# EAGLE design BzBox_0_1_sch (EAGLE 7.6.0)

## Sheet 1 of 6: BME280 EnvSense
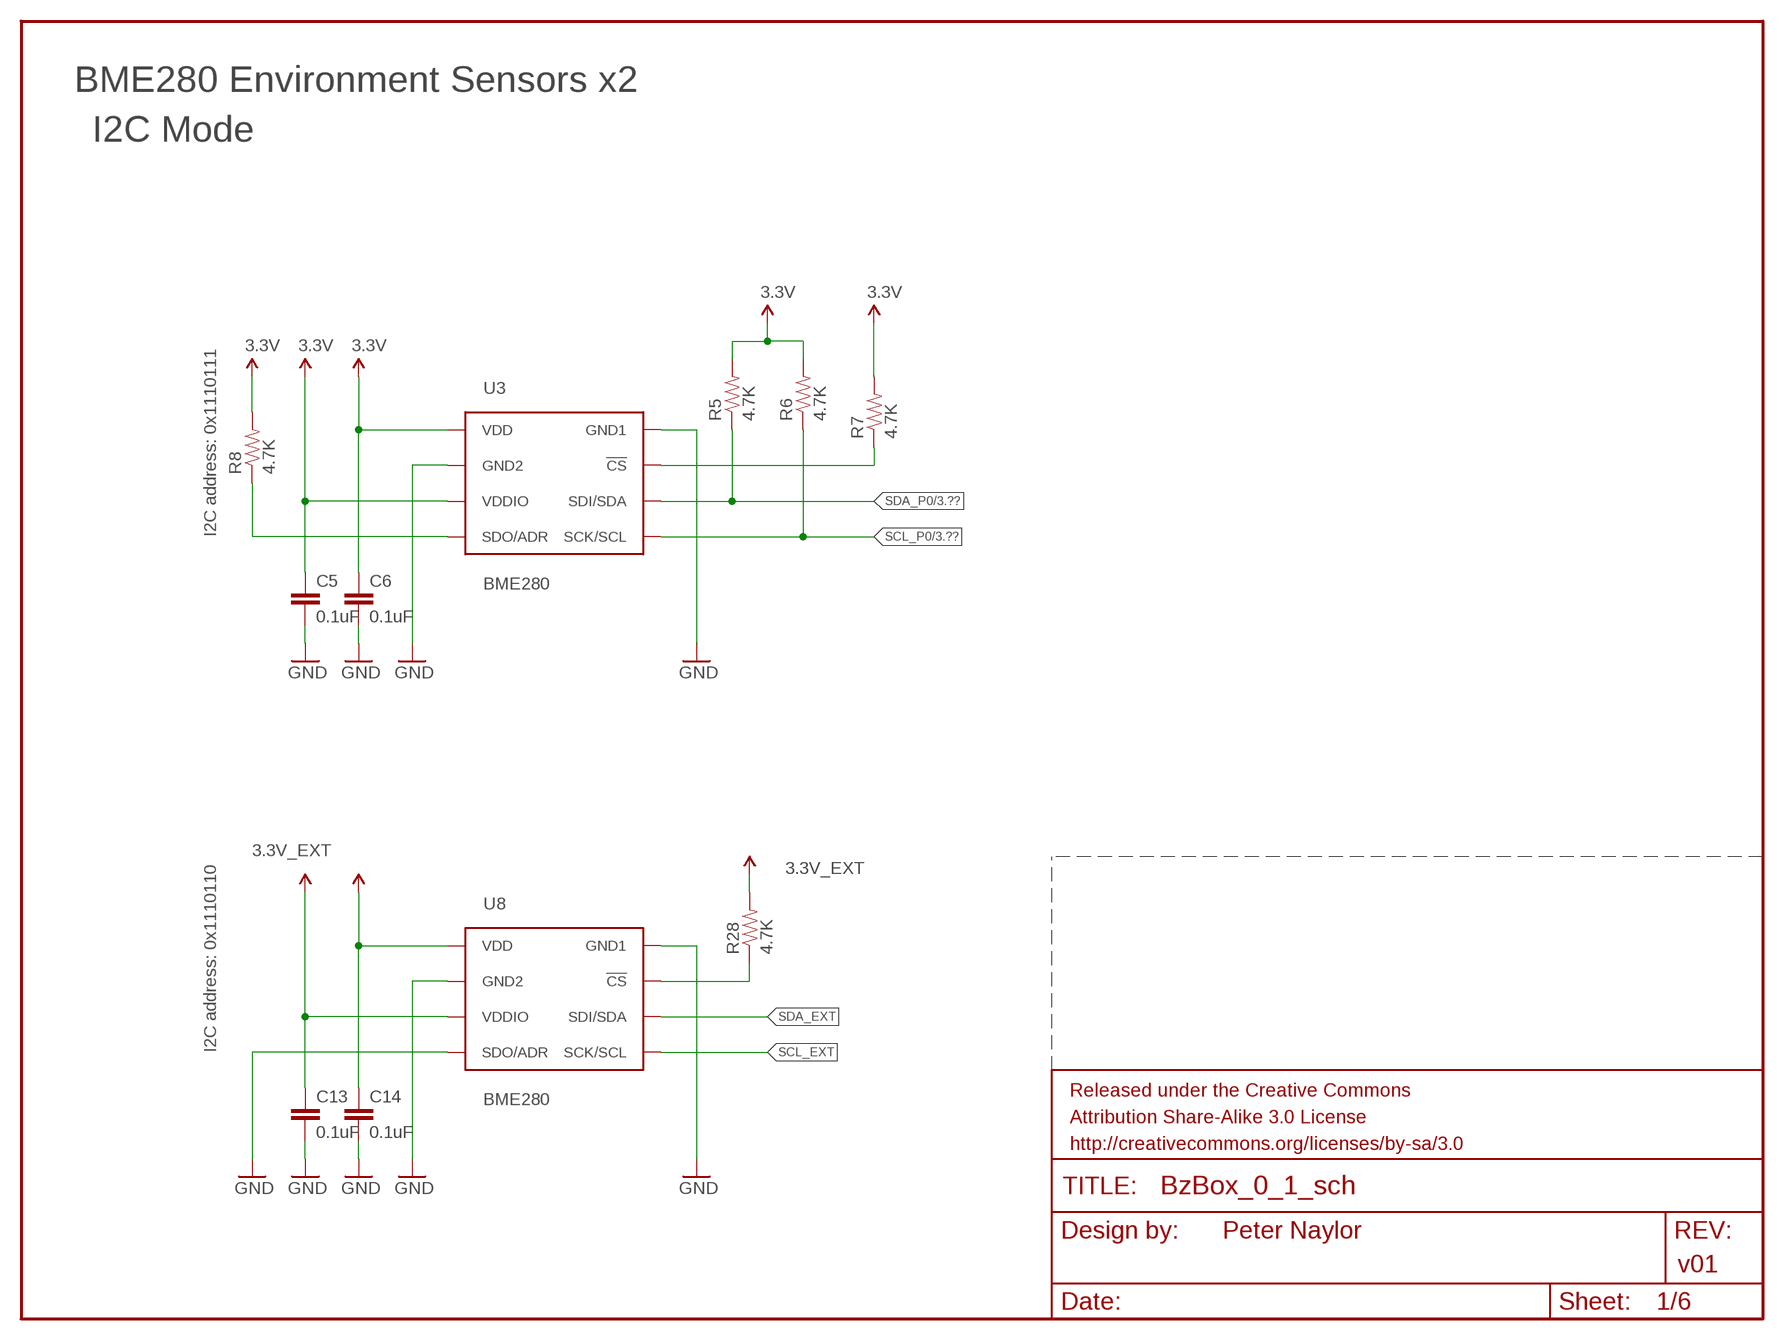
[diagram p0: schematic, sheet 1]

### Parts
C5  0.1uF  0.1UF-25V-5%(0603)  [0603-CAP@1]
C6  0.1uF  0.1UF-25V-5%(0603)  [0603-CAP@1]
C13  0.1uF  0.1UF-25V-5%(0603)  [0603-CAP@1]
C14  0.1uF  0.1UF-25V-5%(0603)  [0603-CAP@1]
R5  4.7K  4.7KOHM-1/10W-1%(0603)  [0603-RES]
R6  4.7K  4.7KOHM-1/10W-1%(0603)  [0603-RES]
R7  4.7K  4.7KOHM-1/10W-1%(0603)  [0603-RES]
R8  4.7K  4.7KOHM-1/10W-1%(0603)  [0603-RES]
R28  4.7K  4.7KOHM-1/10W-1%(0603)  [0603-RES]
U3  BME280  [BME280_LGA]
U8  BME280  [BME280_LGA]

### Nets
3.3V: C5.1 C6.1 R5.2 R6.2 R7.2 R8.2 U3.P$6(VDDIO) U3.P$8(VDD) ; also sheet 4,5,6
3.3V_EXT: C13.1 C14.1 R28.2 U8.P$6(VDDIO) U8.P$8(VDD) ; supply symbol labelled 3.3V ; also sheet 2
!CS: R7.1 U3.P$2(!CS)
GND: C5.2 C6.2 U3.P$1(GND1) U3.P$7(GND2) ; also sheet 3,4,5,6
GND_EXT: C13.2 C14.2 U8.P$1(GND1) U8.P$5(SDO/ADR) U8.P$7(GND2) ; supply symbol labelled GND ; also sheet 2
N$3: R28.1 U8.P$2(!CS)
SCL_EXT: U8.P$4(SCK/SCL) ; also sheet 2
SCL_P0: R6.1 U3.P$4(SCK/SCL) ; also sheet 3,5,6
SDA_EXT: U8.P$3(SDI/SDA) ; also sheet 2
SDA_P0: R5.1 U3.P$3(SDI/SDA) ; also sheet 3,5,6
SDO/ADR: R8.1 U3.P$5(SDO/ADR)

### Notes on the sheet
- BME280 Environment Sensors x2
- I2C Mode
- I2C address: 0x1110111
- I2C address: 0x1110110
- Peter Naylor
- v01

## Sheet 2 of 6: ADMP401 uPhone
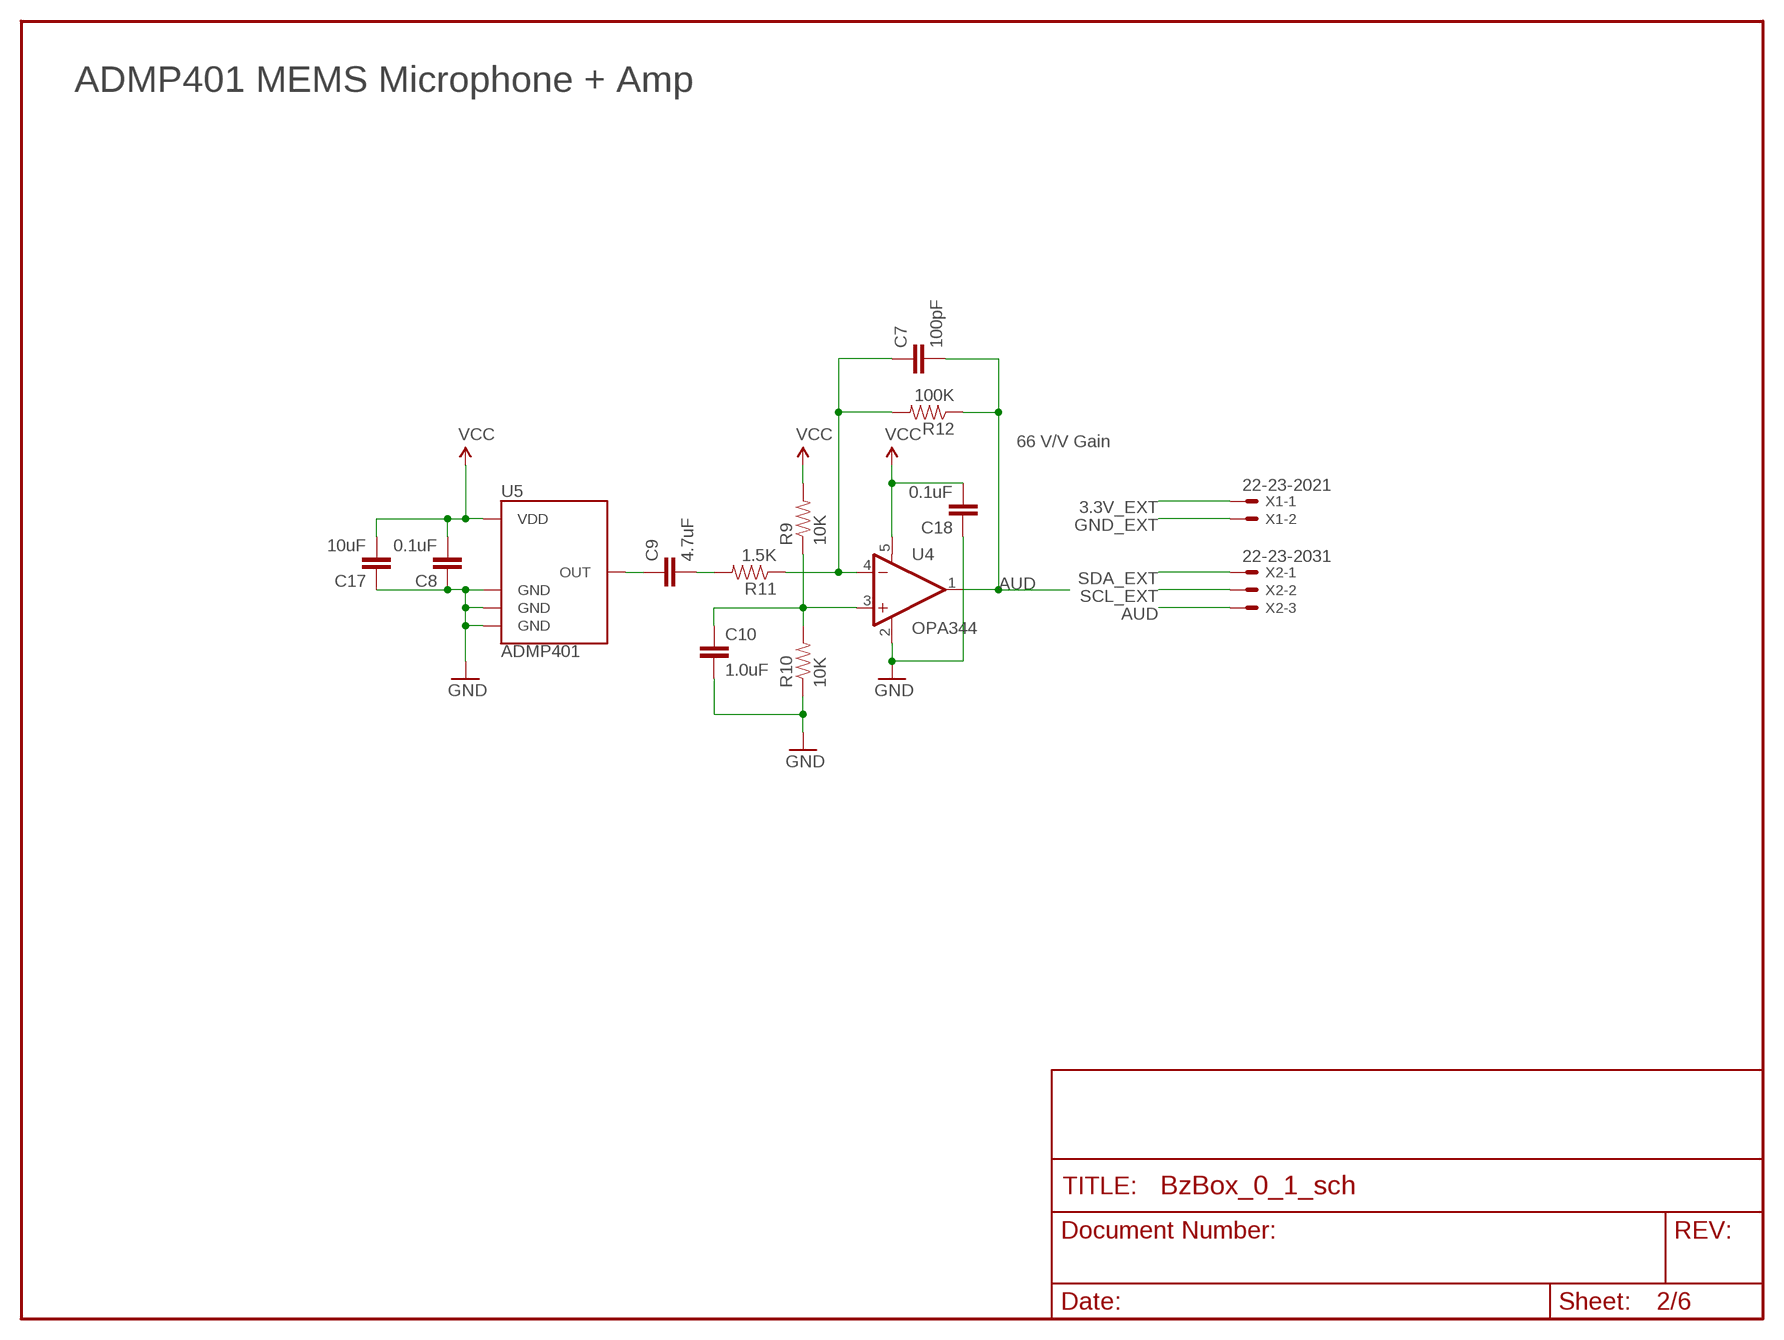
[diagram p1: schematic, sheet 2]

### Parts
C7  100pF  CAP0402-CAP  [0402-CAP]
C8  0.1uF  CAP0402-CAP  [0402-CAP]
C9  4.7uF  CAP0402-CAP  [0402-CAP]
C10  1.0uF  CAP0402-CAP  [0402-CAP]
C17  10uF  CAP0402-CAP  [0402-CAP]
C18  0.1uF  CAP0402-CAP  [0402-CAP]
R9  10K  RESISTOR0402-RES  [0402-RES]
R10  10K  RESISTOR0402-RES  [0402-RES]
R11  1.5K  RESISTOR0402-RES  [0402-RES]
R12  100K  RESISTOR0402-RES  [0402-RES]
U4  OPA344  [SOT23-5]
U5  ADMP401  [ADMP401]
X1  22-23-2021  [22-23-2021]
X2  22-23-2031  [22-23-2031]

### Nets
3.3V_EXT: C8.2 C17.2 C18.2 R9.2 U4.5(V+) U5.5(VDD) X1.1 ; supply symbol labelled VCC ; also sheet 1
AUD: C7.2 R12.1 U4.1(OUT) X2.3
GND_EXT: C8.1 C10.2 C17.1 C18.1 R10.1 U4.2(V-) U5.2(GND) U5.4(GND) U5.6(GND) X1.2 ; supply symbol labelled GND ; also sheet 1
N$9: C9.1 U5.1(OUT)
N$10: C7.1 R11.1 R12.2 U4.4(-IN)
N$11: C9.2 R11.2
N$12: C10.1 R9.1 R10.2 U4.3(+IN)
SCL_EXT: X2.2 ; also sheet 1
SDA_EXT: X2.1 ; also sheet 1

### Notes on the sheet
- ADMP401 MEMS Microphone + Amp
- 66 V/V Gain

## Sheet 3 of 6: Solar-Battery Charger
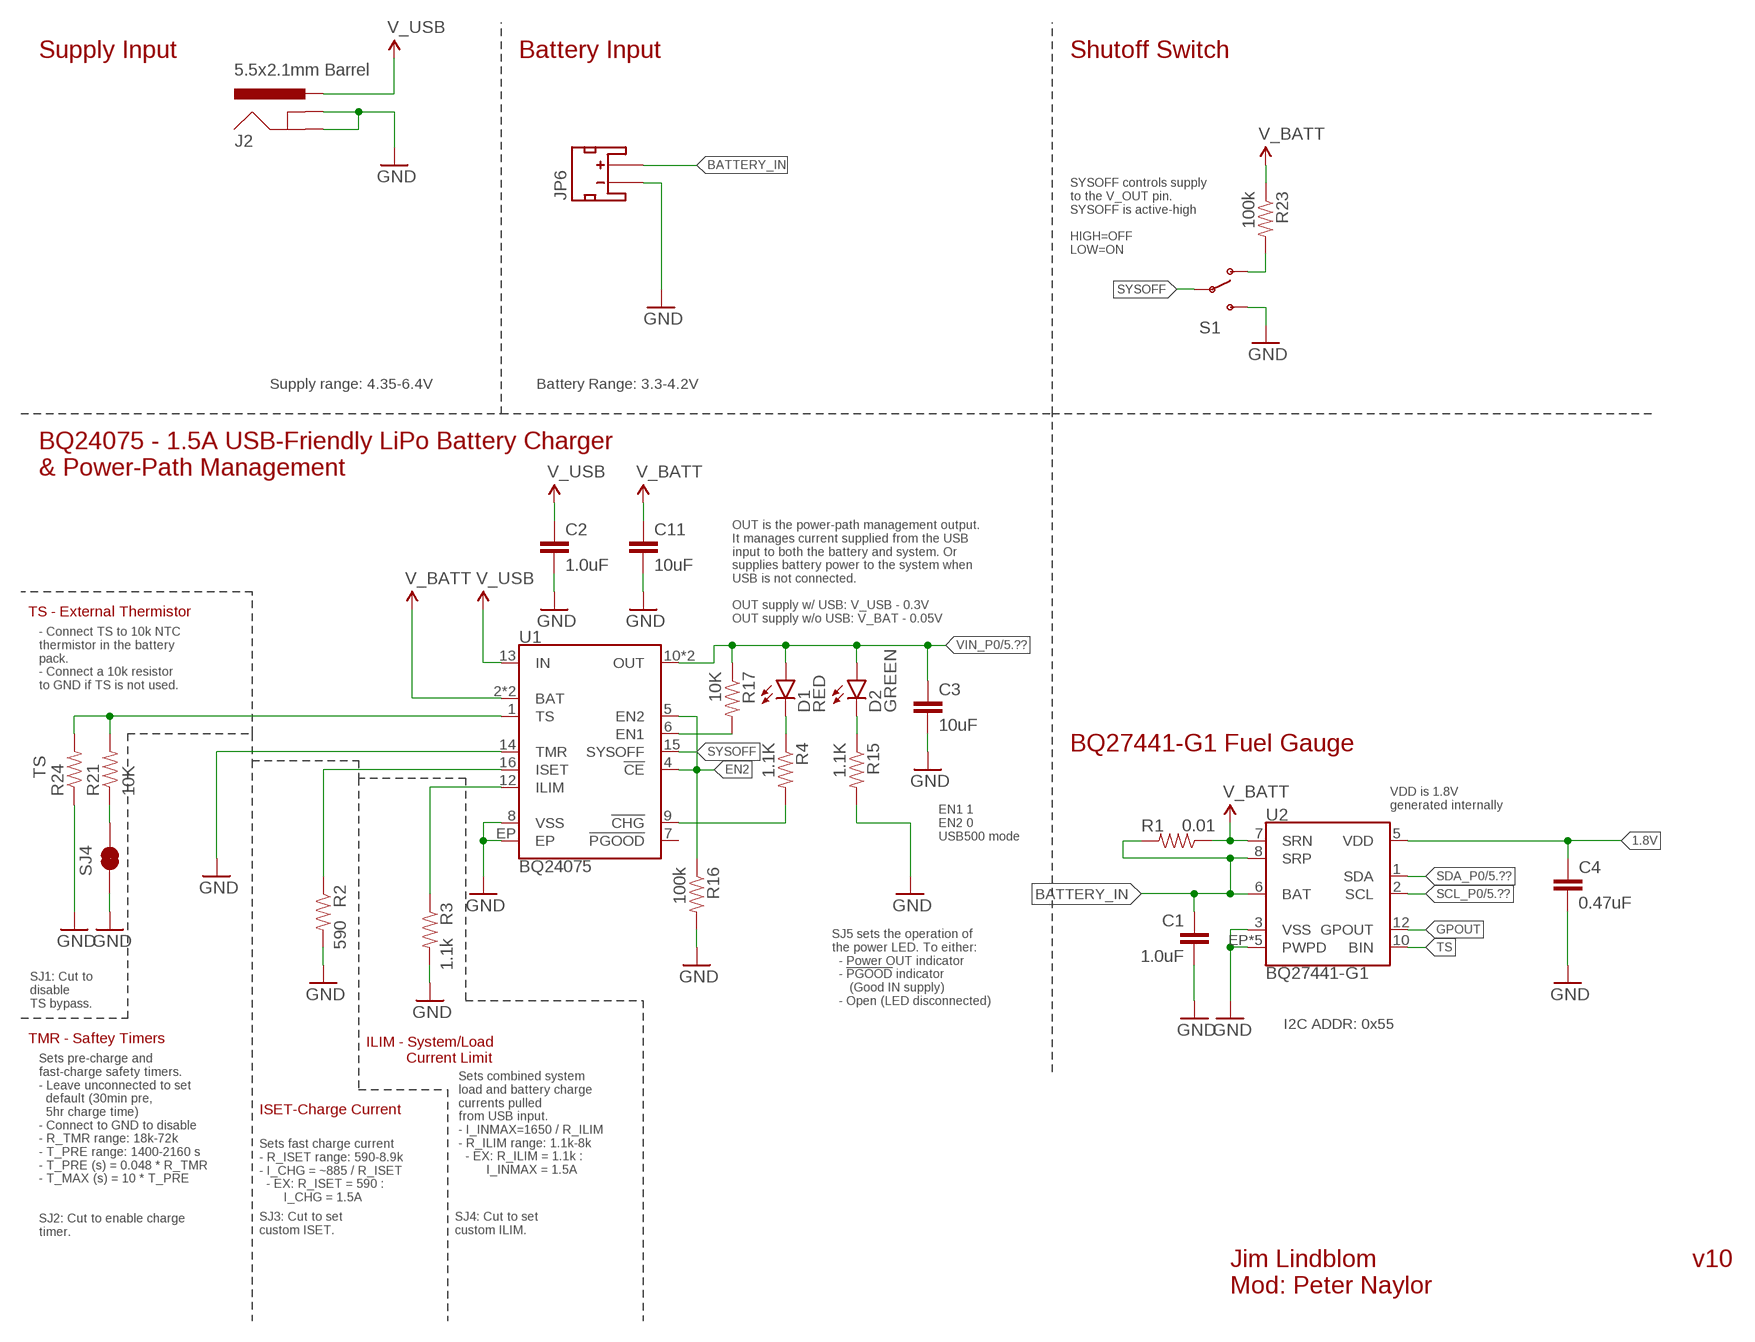
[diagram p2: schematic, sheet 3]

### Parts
C1  1.0uF  1.0UF-16V-10%(0603)  [0603-CAP]
C2  1.0uF  1.0UF50V10%(1206)  [1206-CAP]
C3  10uF  10UF10V10%(0805)  [0805-CAP]
C4  0.47uF  CAP0603-CAP  [0603-CAP]
C11  10uF  10UF10V10%(0805)  [0805-CAP]
D1  RED  LED-BLUE0603  [LED-0603]
D2  GREEN  LED-RED0603  [LED-0603]
J2  5.5x2.1mm Barrel  POWER_JACKSMD  [POWER_JACK_SMD]
JP6  JST_2MM_MALE  [JST-2-SMD]
R1  0.01  RESISTOR1206  [1206]
R2  590  RESISTOR0603-RES  [0603-RES]
R3  1.1k  RESISTOR0603-RES  [0603-RES]
R4  1.1K  180OHM1/10W1%(0603)  [0603-RES]
R15  1.1K  1KOHM-1/10W-1%(0603)  [0603-RES]
R16  100k  100KOHM-1/10W-1%(0603)  [0603-RES]
R17  10K  10KOHM-1/10W-1%(0603)0603  [0603-RES]
R21  10K  10KOHM-1/10W-1%(0603)0603  [0603-RES]
R23  100k  100KOHM-1/10W-1%(0603)  [0603-RES]
R24  TS  RESISTORPTH-1/6W  [1/6W-RES]
S1  SWITCH-SPDT-SMD-A  [SWITCH-SPST-SMD-A]
SJ4  JUMPER-PAD-2-NC_BY_TRACE  [PAD-JUMPER-2-NC_BY_TRACE_YES_SILK]
U1  BQ24075  [PVQFN-N16]
U2  BQ27441-G1  [PDSO-N12]

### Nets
1.8V: C4.1 U2.5(VDD)
!CHG!: R4.2 U1.9(!CHG!)
BATTERY_IN: C1.1 JP6.2(+) R1.2 U2.6(BAT) U2.8(SRP)
EN1: R17.2 U1.6(EN1)
EN2: R16.1 U1.4(!CE!) U1.5(EN2)
GND: C1.2 C2.2 C3.2 C4.2 C11.2 J2.GND(GNDBREAK) J2.P$4(GND) JP6.1(-) R2.2 R3.2 R15.2 R16.2 R24.1 S1.3(S) SJ4.1 U1.8(VSS) U1.14(TMR) U1.EP U2.3(VSS) U2.EP1(PWPD) U2.EP2(PWPD) U2.EP3(PWPD) U2.EP4(PWPD) U2.EP(PWPD) ; also sheet 1,4,5,6
GPOUT: U2.12(GPOUT)
ILIM: R3.1 U1.12(ILIM)
ISET: R2.1 U1.16(ISET)
N$1: D1.C R4.1
N$2: D2.C R15.1
N$6: R23.2 S1.1(O)
N$7: R21.1 SJ4.2
SCL_P0: U2.2(SCL) ; also sheet 1,5,6
SDA_P0: U2.1(SDA) ; also sheet 1,5,6
SYSOFF: S1.2(P) U1.15(SYSOFF)
TS: R21.2 R24.2 U1.1(TS) U2.10(BIN)
V_BATT: C11.1 R1.1 R23.1 U1.2(BAT) U1.3(BAT) U2.7(SRN)
V_SOLAR: C2.1 J2.VIN0(PWR) U1.13(IN) ; supply symbol labelled V_USB
VIN_P0: C3.1 D1.A D2.A R17.1 U1.10(OUT) U1.11(OUT) ; also sheet 5
Unconnected: JP6.NC1(PAD1) JP6.NC2(PAD2) U1.7(!PGOOD!)

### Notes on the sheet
- Supply Input | Battery Input | Shutoff Switch
- SYSOFF controls supply 
  to the V_OUT pin.
  SYSOFF is active-high
  
  HIGH=OFF
  LOW=ON
- Supply range: 4.35-6.4V | Battery Range: 3.3-4.2V
- BQ24075 - 1.5A USB-Friendly LiPo Battery Charger 
  & Power-Path Management
- OUT is the power-path management output.
  It manages current supplied from the USB 
  input to both the battery and system. Or
  supplies battery power to the system when 
  USB is not connected.
  
  OUT supply w/ USB: V_USB - 0.3V
  OUT supply w/o USB: V_BAT - 0.05V
- TS - External Thermistor
- - Connect TS to 10k NTC 
  thermistor in the battery
  pack.
  - Connect a 10k resistor 
  to GND if TS is not used.
- BQ27441-G1 Fuel Gauge
- VDD is 1.8V
  generated internally
- EN1 1
  EN2 0
  USB500 mode
- SJ5 sets the operation of 
  the power LED. To either:
    - Power OUT indicator
    - !PGOOD! indicator 
       (Good IN supply)
    - Open (LED disconnected)
- SJ1: Cut to 
  disable
  TS bypass.
- I2C ADDR: 0x55
- TMR - Saftey Timers
- ILIM - System/Load 
            Current Limit
- Sets pre-charge and
  fast-charge safety timers.
  - Leave unconnected to set
    default (30min pre, 
    5hr charge time)
  - Connect to GND to disable
  - R_TMR range: 18k-72k
  - T_PRE range: 1400-2160 s
  - T_PRE (s) = 0.048 * R_TMR
  - T_MAX (s) = 10 * T_PRE
- Sets combined system
  load and battery charge 
  currents pulled
  from USB input.
  - I_INMAX=1650 / R_ILIM
  - R_ILIM range: 1.1k-8k
    - EX: R_ILIM = 1.1k : 
          I_INMAX = 1.5A
- ISET-Charge Current
- Sets fast charge current
  - R_ISET range: 590-8.9k
  - I_CHG = ~885 / R_ISET
    - EX: R_ISET = 590 : 
         I_CHG = 1.5A
- SJ3: Cut to set
  custom ISET.
- SJ4: Cut to set
  custom ILIM.
- SJ2: Cut to enable charge
  timer.
- Jim Lindblom
  Mod: Peter Naylor
- v10

## Sheet 4 of 6: microSD
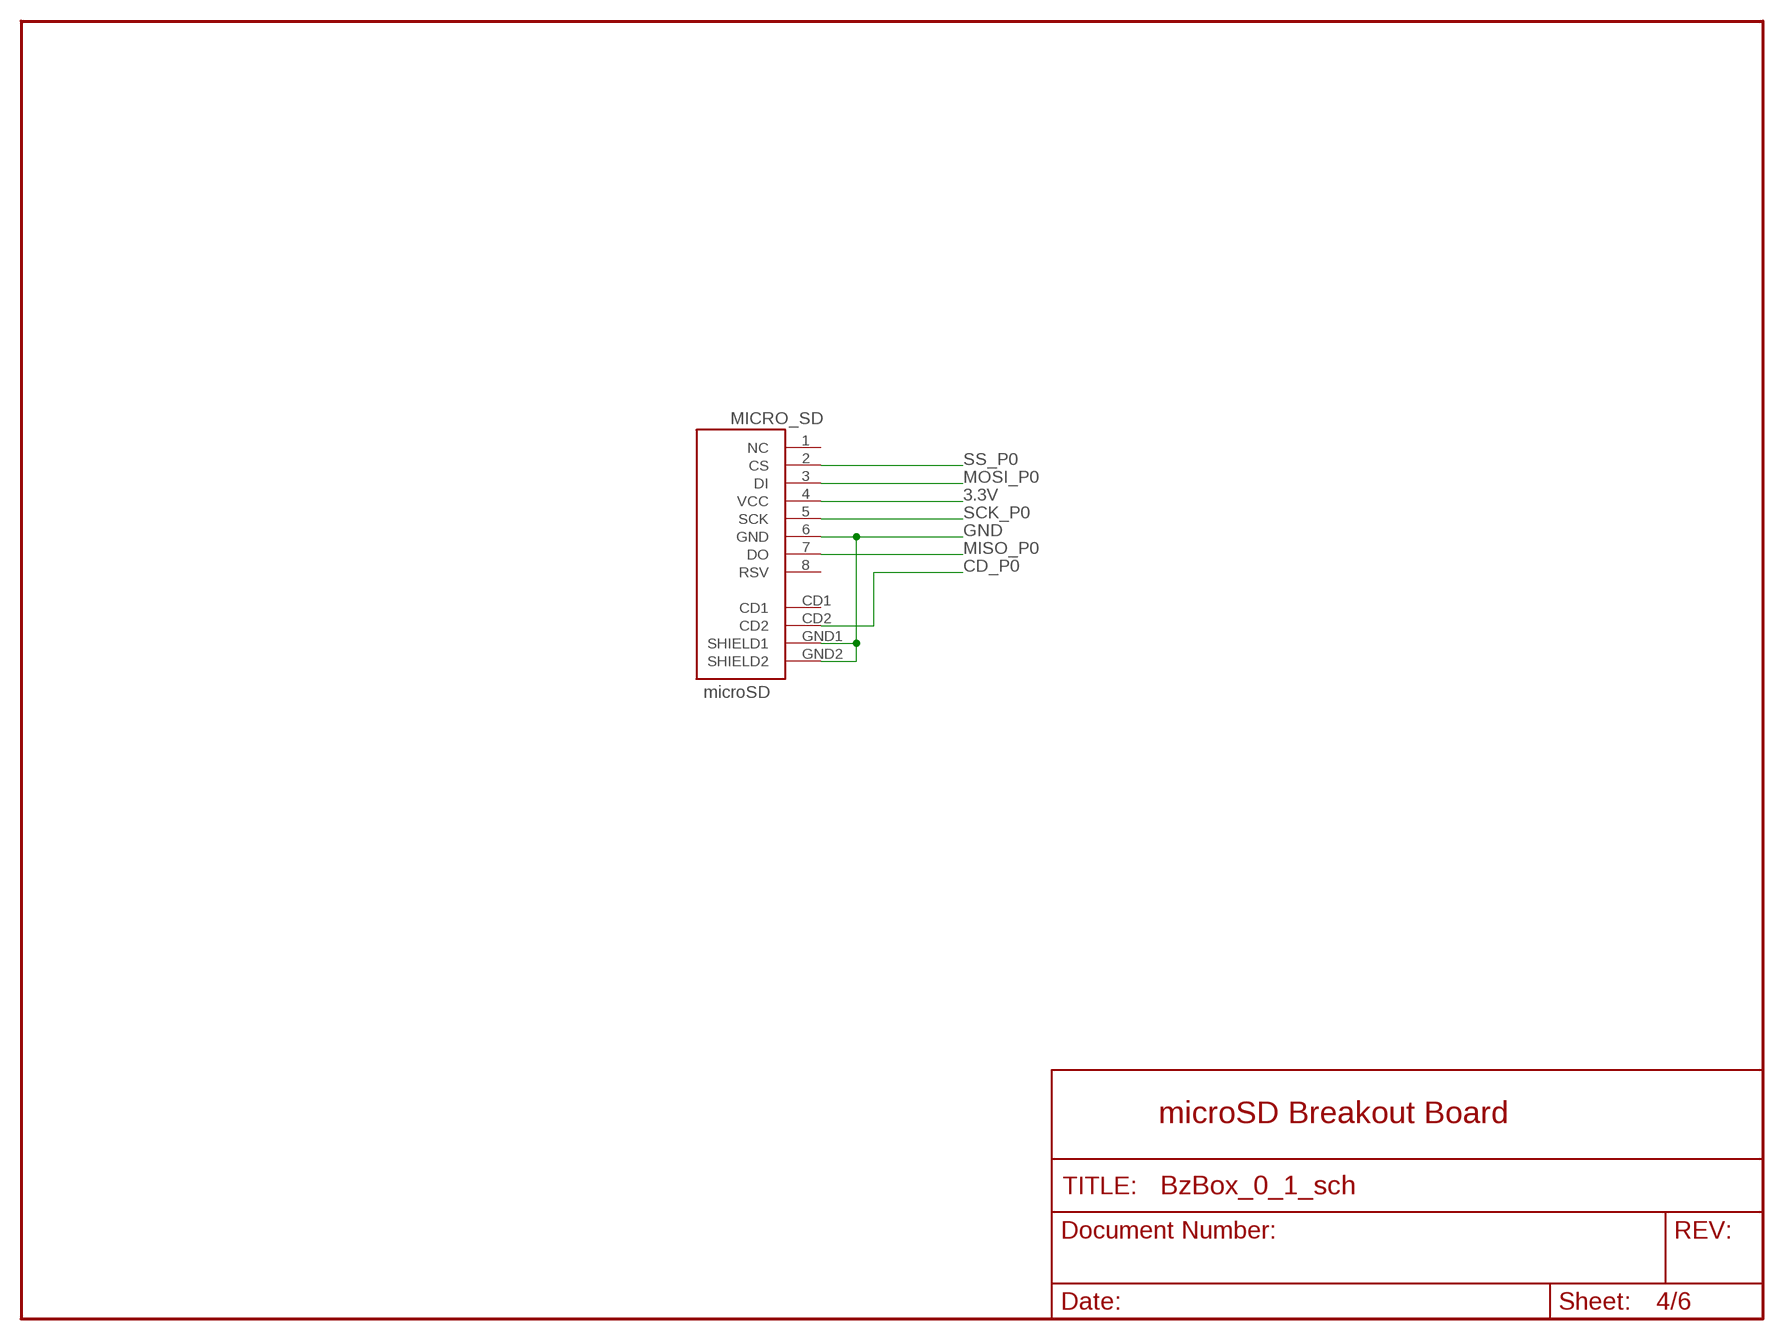
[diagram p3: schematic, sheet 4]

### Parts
MICRO_SD  microSD  USD-SOCKETSMD  [MICRO-SD-SOCKET-PP]

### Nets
3.3V: MICRO_SD.4(VCC) ; also sheet 1,5,6
CD_P0: MICRO_SD.CD2 ; also sheet 5
GND: MICRO_SD.6(GND) MICRO_SD.GND1(SHIELD1) MICRO_SD.GND2(SHIELD2) ; also sheet 1,3,5,6
MISO_P0: MICRO_SD.7(DO) ; also sheet 5
MOSI_P0: MICRO_SD.3(DI) ; also sheet 5
SCK_P0: MICRO_SD.5(SCK) ; also sheet 5
SS_P0: MICRO_SD.2(CS) ; also sheet 5
Unconnected: MICRO_SD.1(NC) MICRO_SD.8(RSV) MICRO_SD.CD1

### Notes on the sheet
- microSD Breakout Board

## Sheet 5 of 6: Main
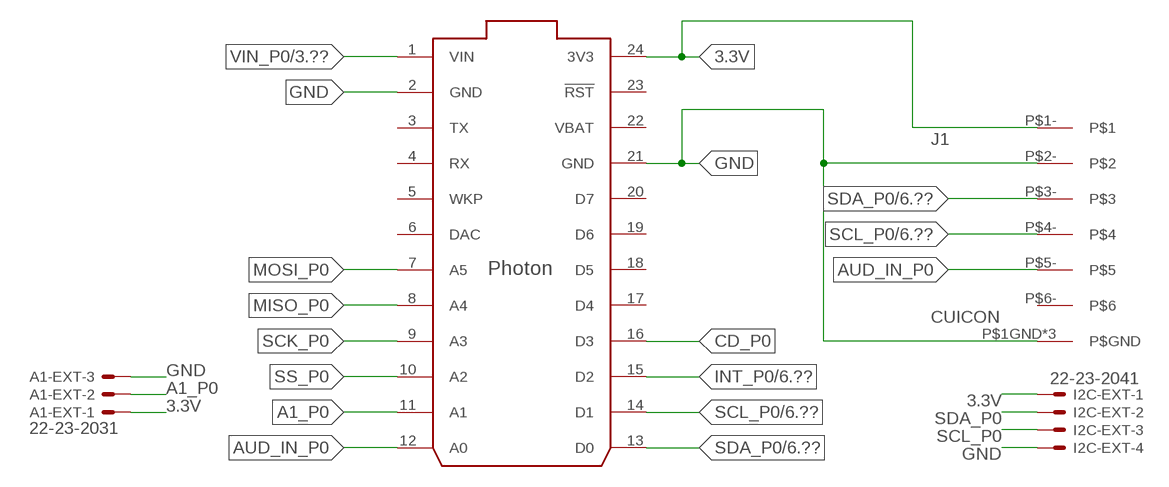
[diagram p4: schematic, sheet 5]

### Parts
A1-EXT  22-23-2031  [22-23-2031]
I2C-EXT  22-23-2041  [22-23-2041]
J1  CUICON  [CUICON]
PHOTON  PHOTON_WITH_HEADERS  [PHOTON]

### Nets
3.3V: A1-EXT.1 I2C-EXT.1 J1.P$1- PHOTON.24(3V3) ; also sheet 1,4,6
A1_P0: A1-EXT.2 PHOTON.11(A1)
AUD_IN_P0: J1.P$5- PHOTON.12(A0)
CD_P0: PHOTON.16(D3) ; also sheet 4
GND: A1-EXT.3 I2C-EXT.4 J1.P$1GND(P$GND) J1.P$2- J1.P$2GND(P$GND) J1.P$3GND(P$GND) PHOTON.2(GND) PHOTON.21(GND) ; also sheet 1,3,4,6
INT_P0: PHOTON.15(D2) ; also sheet 6
MISO_P0: PHOTON.8(A4) ; also sheet 4
MOSI_P0: PHOTON.7(A5) ; also sheet 4
SCK_P0: PHOTON.9(A3) ; also sheet 4
SCL_P0: I2C-EXT.3 J1.P$4- PHOTON.14(D1) ; also sheet 1,3,6
SDA_P0: I2C-EXT.2 J1.P$3- PHOTON.13(D0) ; also sheet 1,3,6
SS_P0: PHOTON.10(A2) ; also sheet 4
VIN_P0: PHOTON.1(VIN) ; also sheet 3
Unconnected: J1.P$6- PHOTON.3(TX) PHOTON.4(RX) PHOTON.5(WKP) PHOTON.6(DAC) PHOTON.17(D4) PHOTON.18(D5) PHOTON.19(D6) PHOTON.20(D7) PHOTON.23(!RST)

## Sheet 6 of 6: ADXL345
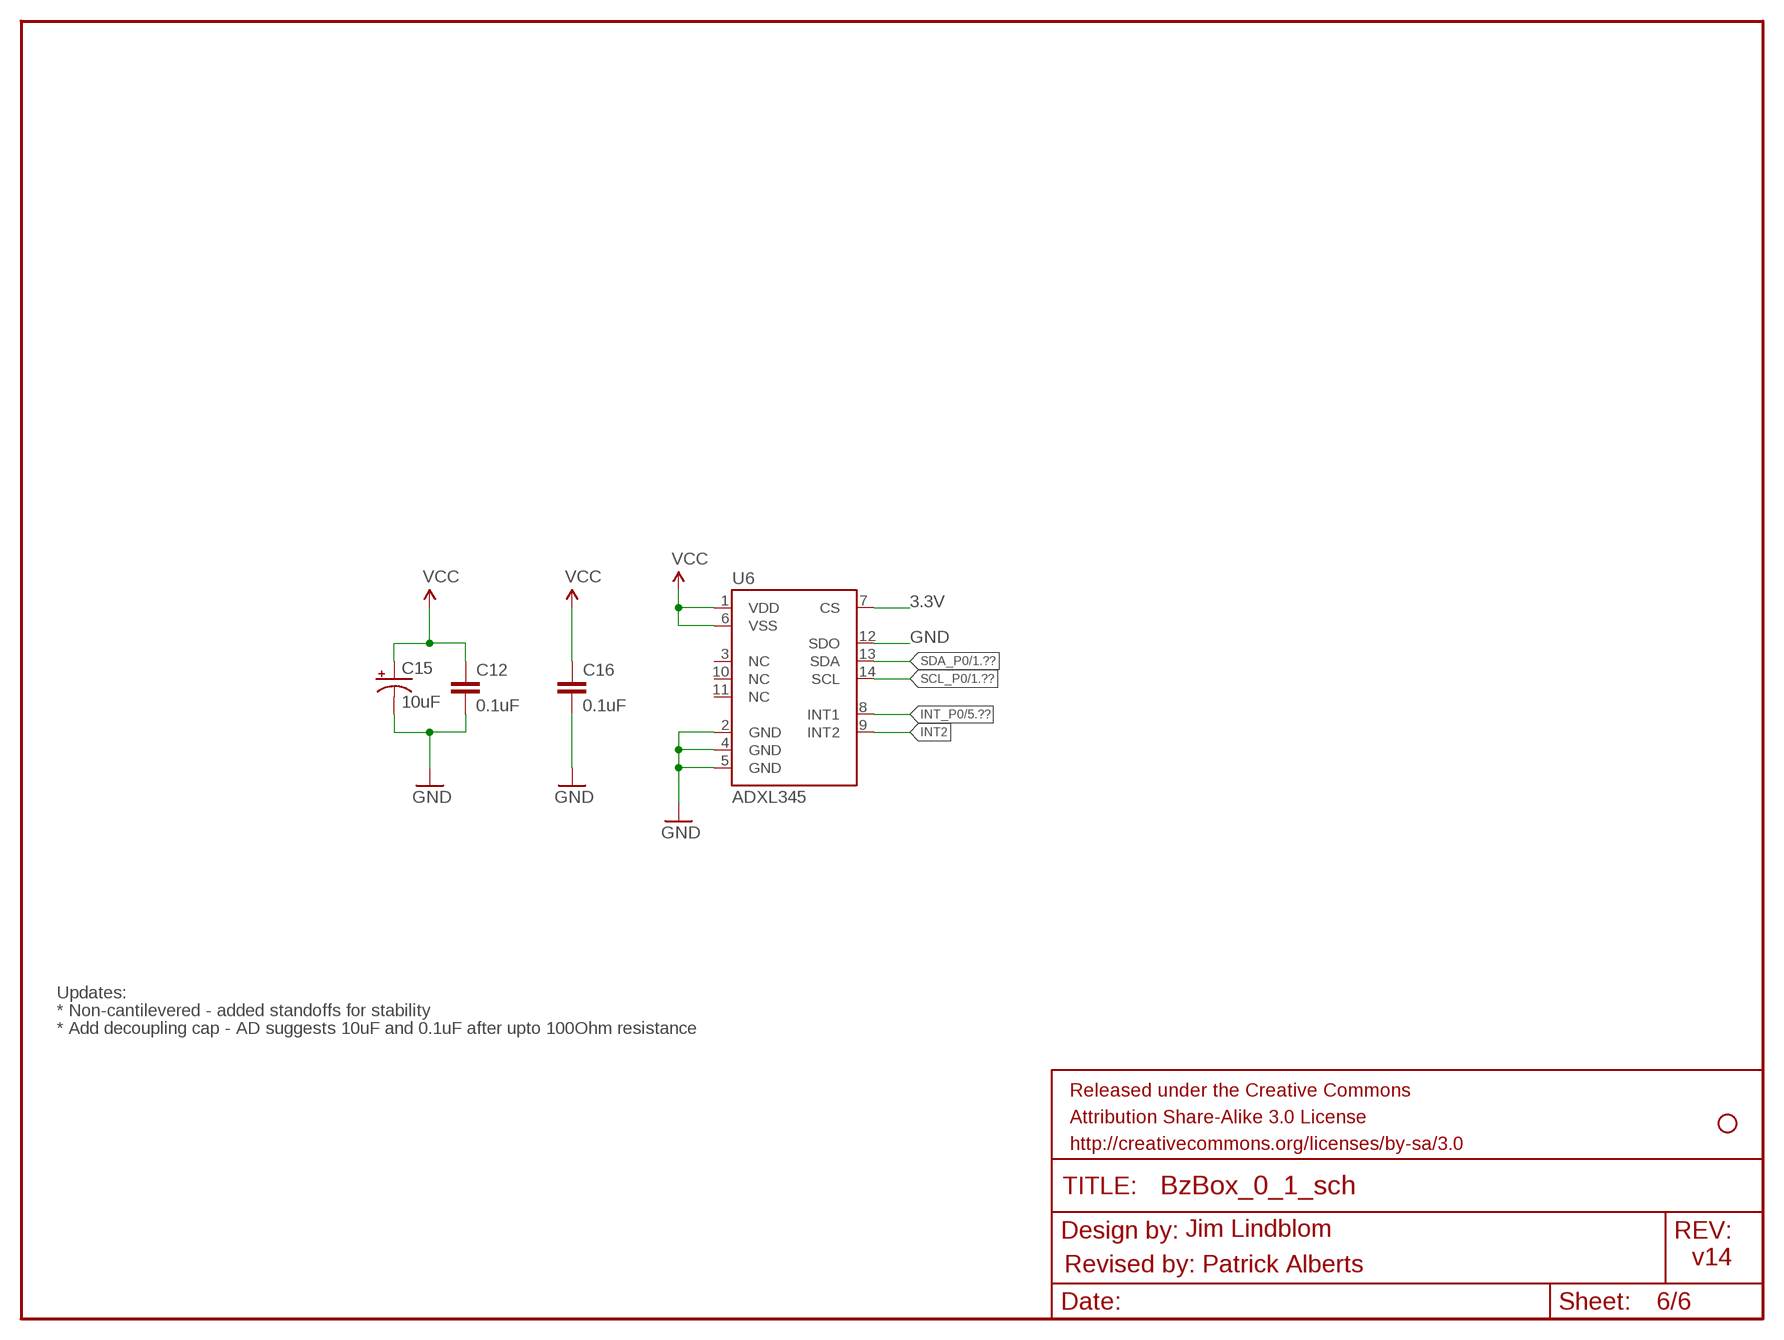
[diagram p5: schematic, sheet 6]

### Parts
C12  0.1uF  CAP0603-CAP  [0603-CAP]
C15  10uF  CAP_POL1206  [EIA3216]
C16  0.1uF  CAP0603-CAP  [0603-CAP]
JP4  STAND-OFF  [STAND-OFF]
U6  ADXL345  ADXL345PATRICK  [LGA14_1:1_PATRICK]

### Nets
3.3V: C12.1 C15.A(+) C16.1 U6.1(VDD) U6.6(VSS) U6.7(CS) ; supply symbol labelled VCC ; also sheet 1,4,5
GND: C12.2 C15.C(-) C16.2 U6.2(GND) U6.4(GND) U6.5(GND) U6.12(SDO) ; also sheet 1,3,4,5
INT2: U6.9(INT2)
INT_P0: U6.8(INT1) ; also sheet 5
SCL_P0: U6.14(SCL) ; also sheet 1,3,5
SDA_P0: U6.13(SDA) ; also sheet 1,3,5
Unconnected: U6.3(NC) U6.10(NC) U6.11(NC)

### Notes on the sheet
- Updates:
- * Non-cantilevered - added standoffs for stability
- * Add decoupling cap - AD suggests 10uF and 0.1uF after upto 100Ohm resistance
- Jim Lindblom
- v14
- Revised by: Patrick Alberts

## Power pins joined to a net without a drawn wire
VBAT: PHOTON.22(VBAT)

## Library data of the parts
A1-EXT X2 = con-molex:22-23-2031: .100" (2.54mm) Center Header - 3 Pin; MF: MOLEX; MPN: 22-23-2031; OC_FARNELL: 1462950; OC_NEWARK: 30C0862
C1 = SparkFun-Capacitors:1.0UF-16V-10%(0603): CAP-00868; PROD_ID: CAP-00868
C2 = SparkFun-Capacitors:1.0UF50V10%(1206): CAP-09822; PROD_ID: CAP-09822
C3 C11 = SparkFun-Capacitors:10UF10V10%(0805): CAP-11330; PROD_ID: CAP-11330
C4 = SparkFun-Capacitors:CAP: Capacitor; PROD_ID: CAP-13216
C5 C6 C13 C14 = SparkFun-Capacitors:0.1UF-25V-5%(0603): CAP-08604; PROD_ID: CAP-08604
C7-C10 C12 C16-C18 = SparkFun:CAP: Capacitor
C15 = SparkFun:CAP_POL: Capacitor Polarized
D1 = SparkFun-LED:LED-BLUE: Blue LEDs for production use; PROD_ID: DIO-08575; VALUE: BLUE
D2 = SparkFun-LED:LED-RED: Assorted Red LEDs; PROD_ID: DIO-00819; VALUE: RED
I2C-EXT = con-molex:22-23-2041: .100" (2.54mm) Center Header - 4 Pin; MF: MOLEX; MPN: 22-23-2041; OC_FARNELL: 1462920; OC_NEWARK: 38C0355
J1 = BzBox:CUICON
J2 = SparkFun-Connectors:POWER_JACK: Power Jack This is the standard 5.5mm barrel jack for power. The PTH is the most common, proven, reliable, footprint. The Slot footprint only works if the mill layer is transmitted to the PCB fab house so be warned. Mating wall wart : TOL-00298 (and others); PROD_ID: CONN-08106; SF_ID: PRT-12748
JP4 = SparkFun:STAND-OFF: Stand Off
JP6 = SparkFun-Connectors:JST_2MM_MALE: Mates to single-cell LiPo batteries. CONN-11443 Now with smashable polarity marks!; BTM_NEG: -; BTM_POS: +; PROD_ID: CONN-11443; TOP_NEG: -; TOP_POS: +
MICRO_SD = SparkFun:USD-SOCKET: microSD Socket Push-push type uSD socket. Schematic element and footprint production proven. Spark Fun Electronics SKU : PRT-00127. tDoc lines correctly indicate media card edge positions when inserting (unlocked, locked, depressed).
PHOTON = Particle-Devices:PHOTON: Particle Photon Wi-Fi through-hole development board footprint
R1 = SparkFun-Resistors:RESISTOR: Resistor; PROD_ID: RES-13218
R2 = SparkFun-Passives:RESISTOR: Resistor; PROD_ID: RES-13217
R3 = SparkFun-Passives:RESISTOR: Resistor; PROD_ID: RES-10447
R4 = SparkFun-Resistors:180OHM1/10W1%(0603): RES-08788; PROD_ID: RES-08788; VALUE: 180
R5-R8 R28 = SparkFun-Resistors:4.7KOHM-1/10W-1%(0603): RES-07857; PROD_ID: RES-07857
R9-R12 = SparkFun:RESISTOR: Resistor
R15 = SparkFun-Resistors:1KOHM-1/10W-1%(0603): RES-07856; PROD_ID: RES-07856; VALUE: 1K
R16 R23 = SparkFun-Resistors:100KOHM-1/10W-1%(0603): RES-07828; PROD_ID: RES-07828
R17 R21 = SparkFun-Resistors:10KOHM-1/10W-1%(0603): RES-00824; PROD_ID: RES-00824
R24 = SparkFun-Resistors:RESISTOR: Resistor
S1 = SparkFun-Electromechanical:SWITCH-SPDT: SPDT Switch Simple slide switch, Spark Fun Electronics SKU : COM-00102 DPDT SMT slide switch, AYZ0202, SWCH-08179; PROD_ID: SWCH-10651
SJ4 = SparkFun-Passives:JUMPER-PAD-2-NC_BY_TRACE
U1 = battery-management-temp:BQ24075; PROD_ID: IC-13219
U2 = battery-management-temp:BQ27441-G1; PROD_ID: IC-13220
U3 U8 = BME280ComponentLibrary:BME280; PROD_ID: IC-13090
U4 = SparkFun:OPA344
U5 = SparkFun:ADMP401
U6 = Testing:ADXL345
X1 = con-molex:22-23-2021: .100" (2.54mm) Center Header - 2 Pin; MF: MOLEX; MPN: 22-23-2021; OC_FARNELL: 1462926; OC_NEWARK: 25C3832

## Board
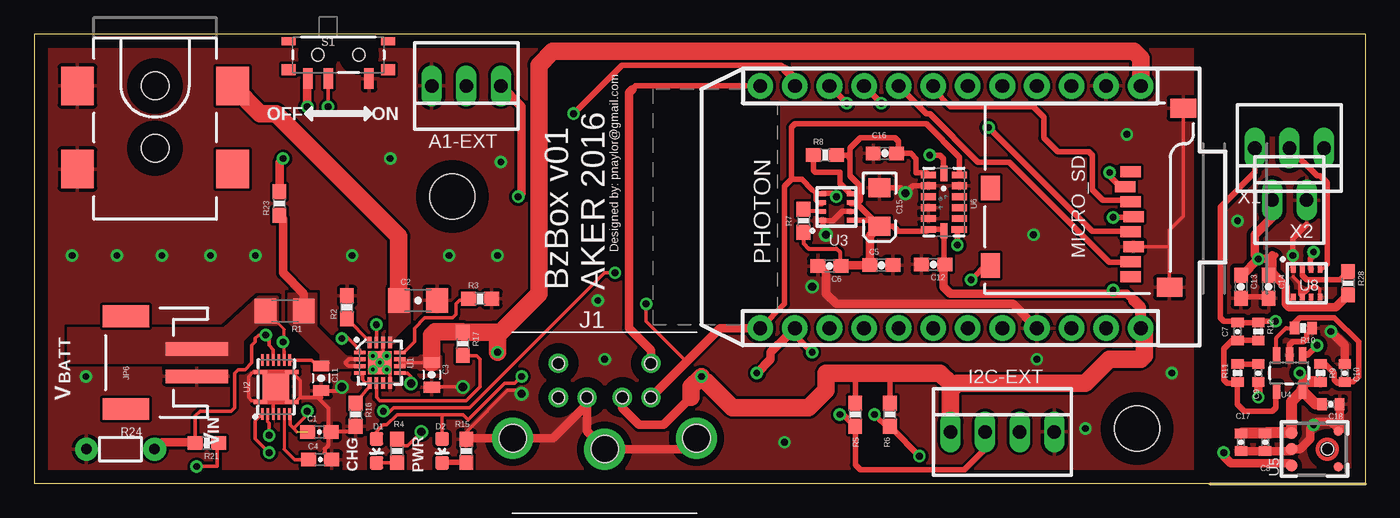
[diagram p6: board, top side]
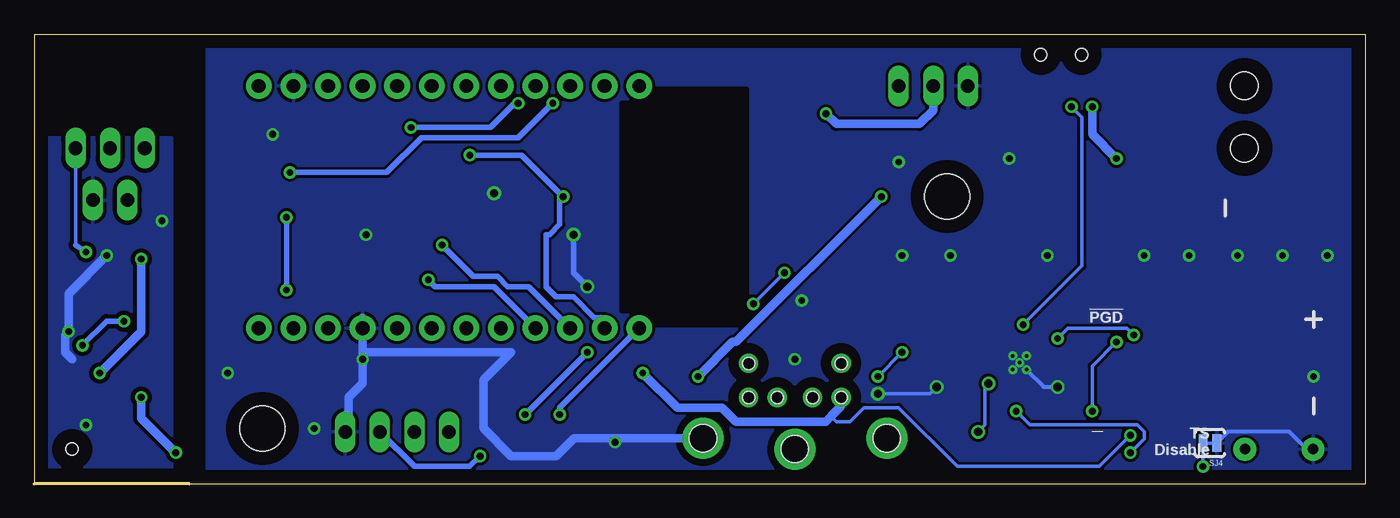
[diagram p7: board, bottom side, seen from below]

Size 97.79 x 33.02 mm. Coordinates in mm from the lower left corner, seen from the top.
Outline: 86.36,0 97.79,0
Outline: 97.79,0 0,0 0,33.02 97.79,33.02 97.79,0
Copper layers (1*16): Top 0.035mm / dielectric 1.5mm / Bottom 0.035mm
Design rules "default": minimum track width 10mil, minimum drill 24mil, track to track 8mil, track to pad 8mil, pad to pad 8mil, via to via 8mil, smd to smd 8mil, copper to edge 40mil, drill to drill 8mil, minimum pad ring 10mil, minimum via ring 8mil, stop-mask expansion 4mil, vias tented up to drill 0mil, thermal gap 10mil

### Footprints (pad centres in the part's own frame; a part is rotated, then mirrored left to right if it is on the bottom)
22-23-2031 = drill 1 long: 1 -2.54,0; 2 0,0; 3 2.54,0
0603-CAP = smd 1.1 x 1: 1 -0.85,0; 2 0.85,0
1206-CAP = smd 1.6 x 1.8: 1 -1.4,0; 2 1.4,0
0805-CAP = smd 0.8 x 1.2: 1 -0.9,0; 2 0.9,0
0603-CAP@1 = smd 1.1 x 1: 1 -0.85,0; 2 0.85,0
0402-CAP = smd 0.7 x 0.9: 1 -0.65,0; 2 0.65,0
EIA3216 = smd 1.4 x 1.6: A 1.4,0; C -1.4,0
LED-0603 = smd 1 x 1: A 0,-0.877; C 0,0.877
22-23-2041 = drill 1 long: 1 -3.81,0; 2 -1.27,0; 3 1.27,0; 4 3.81,0
CUICON = drill 0.9: P$1- -1.3,-3.8; P$2- 1.3,-3.8; P$3- -3.4,-3.8; P$4- 3.4,-3.8; P$5- -3.4,-6.3; P$6- 3.4,-6.3 | drill 2: P$1GND -6.75,-0.8; P$2GND 0,0; P$3GND 6.75,-0.8 | hole 0.9: 1.3,-3.8; -1.3,-3.8; 3.4,-3.8; -3.4,-3.8; 3.4,-6.3; -3.4,-6.3 | hole 2: 0,0; 6.75,-0.8; -6.75,-0.8
POWER_JACK_SMD = smd 2.8 x 2.4: GND 0,-5.7; P$4 6.1,-5.7; VIN0 0,5.7; VIN1 6.1,5.7 | hole 2.032: 0,0; 4.572,0
STAND-OFF = hole 3.302: 0,0
JST-2-SMD = smd 1 x 4.6: 1 -1,-3.7; 2 1,-3.7 | smd 1.6 x 3.4: NC1 -3.4,1.5; NC2 3.4,1.5
MICRO-SD-SOCKET-PP = smd 0.8 x 1.5: 1 -8.94,10.7; 2 -7.84,10.3; 3 -6.74,10.7; 4 -5.64,10.9; 5 -4.54,10.7; 6 -3.44,10.9; 7 -2.34,10.7; 8 -1.24,10.7 | smd 1.8 x 1.4: CD1 -7.75,0.4; CD2 -2.05,0.4 | smd 1.4 x 1.9: GND1 -13.6,14.55; GND2 -0.45,13.55
PHOTON = drill 1.016 pad 1.88: 1 1.27,33.02; 2 1.27,30.48; 3 1.27,27.94; 4 1.27,25.4; 5 1.27,22.86; 6 1.27,20.32; 7 1.27,17.78; 8 1.27,15.24; 9 1.27,12.7; 10 1.27,10.16; 11 1.27,7.62; 12 1.27,5.08; 13 19.05,5.08; 14 19.05,7.62; 15 19.05,10.16; 16 19.05,12.7; 17 19.05,15.24; 18 19.05,17.78; 19 19.05,20.32; 20 19.05,22.86; 21 19.05,25.4; 22 19.05,27.94; 23 19.05,30.48; 24 19.05,33.02
1206 = smd 1.6 x 1.8: 1 -1.4,0; 2 1.4,0
0603-RES = smd 1.1 x 1: 1 -0.85,0; 2 0.85,0
0402-RES = smd 0.7 x 0.9: 1 -0.65,0; 2 0.65,0
1/6W-RES = drill 0.762 pad 1.676: 1 -2.5,0; 2 2.5,0
SWITCH-SPST-SMD-A = smd 0.7 x 1.5: 1 -2.25,-1.75; 2 -0.75,-1.75; 3 2.25,-1.75 | smd 1 x 0.6: GND1 -3.65,1; GND3 3.65,1 | smd 1 x 0.8: GND2 -3.65,-1.1; GND4 3.65,-1.1 | hole 0.9: -1.5,0; 1.5,0
PAD-JUMPER-2-NC_BY_TRACE_YES_SILK = smd 0.635 x 1.27: 1 -0.508,0; 2 0.508,0
PVQFN-N16 = smd 0.28 x 0.85: 1 -0.75,-1.475; 2 -0.25,-1.475; 3 0.25,-1.475; 4 0.75,-1.475; 9 0.75,1.475; 10 0.25,1.475; 11 -0.25,1.475; 12 -0.75,1.475 | smd 0.85 x 0.28: 5 1.475,-0.75; 6 1.475,-0.25; 7 1.475,0.25; 8 1.475,0.75; 13 -1.475,0.75; 14 -1.475,0.25; 15 -1.475,-0.25; 16 -1.475,-0.75 | smd 1.7 x 1.7: EP 0,0
PDSO-N12 = smd 0.2 x 0.85: 1 -1,-1.975; 2 -0.6,-1.975; 3 -0.2,-1.975; 4 0.2,-1.975; 5 0.6,-1.975; 6 1,-1.975; 7 1,1.975; 8 0.6,1.975; 9 0.2,1.975; 10 -0.2,1.975; 11 -0.6,1.975; 12 -1,1.975 | smd 1.95 x 1.95: EP 0,0 | smd 1 x 0.25: EP1 -1.15,1.1; EP2 -1.15,-1.1; EP3 1.15,-1.1; EP4 1.15,1.1
BME280_LGA = smd 0.5 x 0.35: P$1 1.025,0.975; P$2 1.025,0.325; P$3 1.025,-0.325; P$4 1.025,-0.975; P$5 -1.025,-0.975; P$6 -1.025,-0.325; P$7 -1.025,0.325; P$8 -1.025,0.975
SOT23-5 = smd 0.55 x 1.2: 1 -0.95,-1.3; 2 0,-1.3; 3 0.95,-1.3; 4 0.95,1.3; 5 -0.95,1.3
ADMP401 = smd 0.9 x 0.9: 1 -1.2,2.62; 5 1.2,2.62; 6 0,2.62 | smd 0.7 x 0.7: 2 1.3,-0.8; 4 -1.3,-0.8 | hole 0.9: 0,0
LGA14_1:1_PATRICK = smd 0.5 x 1.124: 1 2,1.138; 2 1.2,1.138; 3 0.4,1.138; 4 -0.4,1.138; 5 -1.2,1.138; 6 -2,1.138; 8 -2,-1.13; 9 -1.2,-1.138; 10 -0.4,-1.138; 11 0.4,-1.138; 12 1.2,-1.138; 13 2,-1.138 | smd 1.124 x 0.5: 7 -2.1,0; 14 2.1,0
22-23-2021 = drill 1 long: 1 -1.27,0; 2 1.27,0

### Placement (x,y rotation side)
A1-EXT  31.75,29.21 180 top
C1  20.95,3.81 0 top
C2  28.19,13.46 0 top
C3  29.21,8 270 top
C4  21.02,1.78 0 top
C5  62.23,16.05 0 top
C6  58.42,15.99 180 top
C7  88.39,11.18 90 top
C8  90.42,3.05 90 top
C9  89.92,8.13 90 top
C10  96.27,8.13 90 top
C11  21.08,7.75 270 top
C12  66.04,16.1 180 top
C13  88.65,14.48 270 top
C14  90.68,14.48 270 top
C15  62.1,20.32 270 top
C16  62.48,24.26 180 top
C17  88.65,3.05 90 top
C18  95.25,5.84 180 top
D1  25.15,2.41 180 top
D2  29.97,2.41 180 top
I2C-EXT  71.12,3.81 0 top
J1  41.91,2.54 180 top
J2  8.89,29.21 270 top
JP2  STAND-OFF  [STAND-OFF]  81.03,4.06 180 top
JP4  30.73,21.08 180 top
JP6  8.26,8.89 90 top
MICRO_SD  69.85,13.97 270 top
PHOTON  48.26,30.48 270 top
R1  18.41,12.7 180 top
R2  22.99,12.95 90 top
R3  32.77,13.59 0 top
R4  26.67,2.41 90 top
R5  60.33,5.08 90 top
R6  62.87,5.08 90 top
R7  56.52,19.3 270 top
R8  58.1,24.13 0 top
R9  94.49,8.13 270 top
R10  93.22,11.43 180 top
R11  88.39,8.13 90 top
R12  89.92,11.18 270 top
R15  31.75,2.41 90 top
R16  23.62,5.08 270 top
R17  31.5,10.29 270 top
R21  12.7,2.98 180 top
R23  18.03,20.57 90 top
R24  6.35,2.54 0 top
R28  96.52,14.73 270 top
S1  22.35,31.5 0 top
SJ4  11.43,2.98 180 bottom
U1  25.4,8.89 270 top
U2  17.78,7.11 0 top
U3  58.93,20.32 180 top
U4  92.2,8.13 180 top
U5  95,2.54 90 top
U6  66.83,20.68 90 top
U8  93.47,14.73 90 top
X1  92.2,20.83 0 top
X2  92.2,24.64 180 top

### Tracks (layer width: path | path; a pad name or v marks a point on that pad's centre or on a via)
1.8V
  Top 0.203: U2.5 18.38,2.55
  Top 0.254: C4.1 19.15,1.78 18.38,2.55
3.3V  (via drill 0.5)
  Top 0.254: 43.18,6.37 J1.P$1-
  Top 0.305: R7.2 56.52,17.65 56.9,17.27 58.93,17.27 59.18,17.02 59.18,16.07 C6.1
  Top 0.406: R5.2 60.33,7.75 59.94,8.13 | 57.78,7.75 58.17,8.13 | R6.2 62.87,8 62.99,8.13 | R8.2 59.69,24.13 59.94,23.88 | 59.94,23.88 59.94,22.61 60.71,21.84 60.71,20.83 60.45,20.57 | U3.P$6 60.02,20.57 60.45,20.57 | 60.45,20.57 C15.A | U3.P$8 61.68,19.34 C15.A | 59.94,23.88 59.94,24.64 60.71,25.4 63.25,25.4 63.5,25.15 63.5,24.42 C16.1 64.39,24.26 64.77,23.88 64.77,22.83 65.53,22.83 U6.1 | v79.25,19.56 80.52,19.56 MICRO_SD.4 | v79.25,14.22 79.25,13.97 | C15.A 63.12,18.92 63.5,18.54 65.56,18.54 U6.6 66.73,18.68 U6.7 66.83,16.17 C12.1
  Top 0.61: C15.A 61.38,18.2 C5.1 59.33,16.05 C6.1 | 80.77,13.46 80.26,13.97 79.25,13.97 67.31,13.97 66.8,14.48 66.8,16.02 C12.1 | 43.18,6.37 43.18,5.59 44.45,4.32 46.23,4.32 48.26,6.35 | A1-EXT.1 35.81,27.69 35.81,21.34 v35.56,21.08 | v49.02,7.87 49.4,7.49
  Top 0.813: PHOTON.24 81.28,12.95 80.77,13.46
  Top 1.27: I2C-EXT.1 67.31,6.86 | 67.31,6.86 67.82,7.37 77.22,7.37 78.99,9.14 81.28,9.14 81.53,9.4 81.53,11.18 PHOTON.24 | 67.31,6.86 67.31,7.37 66.55,8.13 62.99,8.13 59.94,8.13 58.17,8.13 58.17,6.86 56.9,5.59 51.31,5.59 49.4,7.49 | 48.26,6.35 48.26,7.11 v49.02,7.87
  Bottom 0.406: v79.25,14.22 v79.25,19.56
  Bottom 0.61: v35.56,21.08 46.23,10.41 46.48,10.41 v49.02,7.87
3.3V_EXT  (via drill 0.5)
  Top 0.254: 91.95,13.21 92,13.21 U8.P$8 | 93.98,12.95 93.8,13.14 U8.P$6
  Top 0.406: 91.19,16.76 90.93,16.76
  Top 0.61: 90.93,16.76 90.93,16.51 | 90.93,16.51 90.93,15.58 C14.1 90.93,15.49 91.95,14.48 91.95,13.21 92.2,12.95 93.98,12.95 95.59,12.95 R28.2 | v92.96,8.13 93.22,7.87 93.22,7.37 93.22,7.11 93.15,7.05 | v89.92,16.51 90.93,16.51 | X1.1 90.93,19.56 89.66,18.29 89.66,16.76 v89.92,16.51 | C13.1 88.73,15.33 v89.92,16.51
  Top 0.813: R9.2 93.33,7.48 93.22,7.37 | C18.2 94.14,5.84 U4.5 | U4.5 93.15,7.05 | U4.5 92.38,6.05 U5.5 90.47,3.74 C8.2 C17.2
  Bottom 0.61: v89.92,16.51 89.92,11.18 v92.96,8.13
!CHG!  (via drill 0.6)
  Top 0.254: v27.69,7.37 27.69,7.87 27.43,8.13 26.92,8.13 U1.9 | R4.2 27.18,2.79 27.43,2.79 v28.45,3.81
  Bottom 0.254: v27.69,7.37 27.94,7.11 27.94,4.32 v28.45,3.81
!CS
  Top 0.305: U3.P$2 56.67,20 R7.1
A1_P0  (via drill 0.5)
  Top 0.406: 55.12,30.48 54.86,30.73 43.18,30.73 v39.62,27.18
  Top 0.61: PHOTON.11 55.88,29.72 55.12,30.48
  Bottom 0.61: A1-EXT.2 31.75,27.43 32.77,26.42 38.86,26.42 v39.62,27.18
AUD  (via drill 0.5)
  Top 0.406: U4.1 93.5,9.43 v94.23,10.16 | v91.19,11.94 89.92,11.94 R12.1 C7.2 88.39,11.94 87.38,11.94 87.12,12.19 87.12,20.32 89.66,22.86 X2.3
  Bottom 0.406: v91.19,11.94 92.46,11.94 v94.23,10.16
AUD_IN_P0
  Top 0.406: PHOTON.12 44.2,29.21 43.94,28.96
  Top 0.61: 43.94,28.96 43.69,28.7 43.69,11.43 45.31,9.81 J1.P$5-
BATTERY_IN  (via drill 0.5)  (1 unrouted)
  Top 0.203: U2.8 18.38,10.41 18.38,11.34 R1.2
  Top 0.254: 19.3,3.81 19.05,4.06 | 19.05,4.06 18.8,4.32 18.8,5.12 U2.6 | U2.8 18.38,9.74 | 19.05,4.06 20.07,5.08 v20.07,5.33 | v18.29,10.41 18.38,10.41
  Bottom 0.254: v20.07,5.33 20.07,8.64 v18.29,10.41
  pour Top (isolate 0.203, no thermals): 2.54,11.43 13.97,11.43 16.51,13.72 17.84,13.72 17.84,11.68 16.51,11.68 15.3,10.48 15.3,8.89 2.54,8.89
CD_P0  (via drill 0.5)
  Top 0.406: v68.83,14.99 70.1,16.26 MICRO_SD.CD2
  Bottom 0.406: v68.83,14.99 68.33,14.48 64.01,14.48 PHOTON.16
EN1
  Top 0.254: U1.6 25.15,6.35 25.4,6.1 31.75,6.1 32.77,7.11 32.77,9.14 32.51,9.4 31.5,9.4 R17.2 31.24,9.18
EN2
  Top 0.254: R16.1 24.38,6.86 24.64,7.11 24.64,7.37 U1.5 24.34,7.42 24.13,7.62 24.13,7.93 U1.4
GND  (via drill 0.25, 0.5, 0.6)
  Top 0.203: U2.3 17.58,4.96
  Top 0.254: MICRO_SD.GND1 84.4,19.63 83.4,18.63 83.4,17.4 | 83.4,17.4 MICRO_SD.GND2 | MICRO_SD.6 83.39,17.41 83.4,17.4 | U2.EP1 16.09,8.21 15.75,7.87 15.75,6.35 16,6.1 16.55,6.1 U2.EP2 17.5,6.01 17.58,6.1 | U2.EP4 19.56,7.58 19.56,6.35 19.22,6.01 U2.EP3 17.92,6.01 17.58,6.35 | 31.83,3.34 31.83,3.89 34.8,6.86 35.56,6.86 v35.81,6.6 | v31.5,7.11 29.21,7.11 C3.2 | U2.3 17.58,6.1 | 17.58,6.1 17.58,6.35 | 17.58,6.35 17.58,6.55 17.53,6.6 17.53,6.86 U2.EP | U1.14 25.65,9.64 v25.9,9.39 | U1.8 26.15,8.14 v25.9,8.39
  Top 0.305: 19.56,6.35 20.83,6.35 | 20.83,6.35 21.09,6.35 C11.2 22.34,6.85 v22.61,7.11 | R16.2 23.62,3.81 C1.2 21.59,3.81 | 21.59,3.81 21.59,5.59 20.83,6.35 | 21.59,3.81 21.59,2.79 21.34,2.54 21.34,2.29 21.84,1.78 C4.2
  Top 0.406: C15.C 63.62,21.72 v64.01,21.34 64.55,21.88 U6.2 | U3.P$7 59.37,20 58.67,19.3 57.94,19.3 | 57.94,19.3 U3.P$1 | 57.94,19.3 57.94,18.51 v58.17,18.29
  Top 0.61: J1.P$2- 40.61,5.84 | 40.61,5.84 40.61,3.84 J1.P$2GND 47.86,2.54 J1.P$1GND | 40.61,5.84 38.11,3.34 J1.P$3GND 31.83,3.34 R15.2 | 58.17,15.49 58.17,13.97 58.93,13.21 71.88,13.21 PHOTON.21
  Bottom 0.254: v35.81,6.6 32,6.6 v31.5,7.11
  Bottom 0.305: R24.1 4.32,2.54 5.59,3.81 10.1,3.81 SJ4.1 | v22.61,7.11 23.62,7.11 v24.9,8.39
  Bottom 0.406: v58.17,18.29 58.17,15.49 v57.15,14.48
  Bottom 0.61: 73.66,9.65 PHOTON.21 73.66,12.19 | 73.66,9.65 v73.66,9.14 73.66,7.37 74.68,6.35 74.68,4.06 I2C-EXT.4 | J1.P$1GND 58.13,3.34 59.44,2.03 62.74,2.03 64.77,4.06 64.77,7.62 62.74,9.65 73.66,9.65
  other vias: 25.4,8.89 24.9,9.39 2.79,16.76 6.1,16.76 9.4,16.76 12.95,16.76 16.26,16.76 3.81,7.87 23.37,16.76 26.16,23.88 30.48,16.76 34.04,16.76 73.41,18.29 83.57,8.13 80.26,25.65 55.12,3.05 41.91,9.14 41.4,13.46 77.22,4.06 34.29,23.62
  pour Top (isolate 0.203, rank 6): 0,0 85.09,0 85.09,33.02 0,33.02
  pour Bottom (isolate 0.203, rank 6): 0,0 85.09,0 85.09,33.02 0,33.02
GND_EXT  (via drill 0.5)
  Top 0.254: 92.5,15.2 92.96,14.73 92.96,13.89 U8.P$7 | U8.P$5 94.45,14.27 94.23,14.48 93.73,14.48 93.47,14.22
  Top 0.406: 92.2,10.16 92.46,10.41 93.22,10.41 93.47,10.67 93.47,11.03 R10.1 | 95.38,11.3 95.25,11.43 | 93.47,19.05 92.46,18.03 v92.46,16.76 92.46,16 U8.P$1 | 93.15,13.9 93.47,14.22 | 90.68,13.72 88.65,13.72 C13.2
  Top 0.61: 95.38,11.3 v95.25,11.18 96.27,10.16 C10.2 | C18.1 95.9,3.94 U5.2 95.8,4.03 95.25,4.57 94.23,4.57 v93.98,4.32 93.73,4.06 93.73,3.3 92.96,2.54 U5.6 92.23,2.4 C8.1 C17.1
  Bottom 0.61: v92.46,16.76 95.25,13.97 v95.25,11.18 95.5,10.92 95.5,9.65 95,9.14
  other vias: 88.39,19.3
  pour Top (isolate 0.305): 87.63,25.4 97.79,25.4 97.79,0 87.63,0
  pour Bottom (isolate 0.305): 87.63,25.4 97.79,25.4 97.79,0 87.63,0
ILIM
  Top 0.254: U1.12 27.17,9.64 27.94,10.41 27.94,11.43 28.7,12.19 30.73,12.19 30.99,12.45 30.99,13.21 31.24,13.46 31.79,13.46 R3.1 32,13.5
INT_P0  (via drill 0.5)
  Top 0.406: v67.82,17.53 67.82,18.54 U6.8
  Bottom 0.406: v67.82,17.53 65.53,15.24 63.75,15.24 62.99,14.48 61.47,14.48 PHOTON.15
ISET
  Top 0.254: U1.16 24.65,10.44 R2.1
MISO_P0
  Top 0.406: PHOTON.8 65.53,27.18 65.79,27.18 69.34,23.62 71.63,23.62 78.99,16.26 80.52,16.26 MICRO_SD.7
MOSI_P0
  Top 0.406: MICRO_SD.3 80.52,20.83 78.49,20.83 77.72,21.59 77.72,24.13 77.47,24.38 75.18,24.38 74.17,25.4 74.17,26.92 73.41,27.69 67.31,27.69 66.04,28.96 PHOTON.7
N$1
  Top 0.254: D1.C 26.64,1.54 R4.1
N$2
  Top 0.406: R15.1 30.25,1.56 D2.C
N$3
  Top 0.406: U8.P$2 93.15,15.31 93.47,14.99 95.92,14.99 R28.1
N$6  (via drill 0.5)
  Top 0.61: v20.07,27.69 20.07,29.72 S1.1 | v18.29,23.88 18.03,23.62 R23.2
  Bottom 0.61: v20.07,27.69 20.07,25.65 v18.29,23.88
N$7  (via drill 0.5)
  Top 0.254: R21.1 13.46,2.79 13.46,1.27 v11.94,1.27
  Bottom 0.254: v11.94,1.27 SJ4.2
N$9  (via drill 0.5)
  Top 0.61: v89.92,6.35 C9.1 | v87.38,2.29 87.38,2.03 87.88,1.52 92.2,1.52 U5.1
  Bottom 0.61: v89.92,6.35 89.92,4.83 v87.38,2.29
N$10
  Top 0.406: R12.2 C7.1 88,10.53 87.38,9.91 87.38,7.62 87.63,7.37 88.28,7.37 R11.1 88.39,5.84 88.9,5.33 90.93,5.33 91.19,5.59 91.19,6.76 U4.4
N$11
  Top 0.406: C9.2 R11.2
N$12
  Top 0.305: U4.3 91.25,10.73 91.95,11.43 R10.2
  Top 0.406: R10.2 92.57,11.8 92.96,12.19 95.5,12.19 97.28,10.41 97.28,7.87 96.89,7.48 C10.1 96.15,7.37 95.76,7.37 95.5,7.62 95.5,8.13 94.85,8.78 R9.1
SCK_P0  (via drill 0.5)
  Top 0.406: v62.23,27.94 PHOTON.9 | v70.1,26.16 77.72,18.54 80.52,18.54 MICRO_SD.5
  Bottom 0.406: v62.23,27.94 62.48,27.94 64.26,26.16 v70.1,26.16
SCL_EXT
  Top 0.254: U8.P$4 94.62,15.76 95,16.13
  Top 0.406: 95,16.13 95,22.1 94.49,22.61 94.23,22.61 X2.2
SCL_P0  (via drill 0.5)
  Top 0.203: 17.14,4.57 17.14,5.1 U2.2
  Top 0.254: v17.27,3.56 17.27,4.45 17.14,4.57
  Top 0.406: PHOTON.14 55.88,10.92 v57.15,9.65 | v61.72,5.08 62.74,4.06 R6.1 62.99,4.06 v65.02,2.03 | v58.93,21.08 58.67,21.34 57.91,21.34 U3.P$4 | U6.14 66.8,22.8 66.8,23.88 66.55,24.13 v65.79,24.13
  Top 0.61: 55.88,10.92 55.37,10.92 54.1,9.65 54.1,9.14 v53.09,8.13
  Bottom 0.254: v17.27,3.56 19.56,1.27 29.97,1.27 34.29,5.59 36.83,5.59 37.85,4.57 38.86,4.57 39.24,4.95
  Bottom 0.406: v61.72,5.08 v57.15,9.65 | v65.02,2.03 65.79,1.27 69.85,1.27 I2C-EXT.3 | PHOTON.14 55.88,12.19 56.64,12.19 58.17,13.72 59.44,13.72 60.2,14.48 60.2,18.29 59.94,18.29 59.18,19.05 59.18,20.83 v58.93,21.08 61.98,24.13 v65.79,24.13
  Bottom 0.61: J1.P$4- 38.51,5.69 39.24,4.95 39.62,4.57 46.23,4.57 47.24,5.59 50.55,5.59 v53.09,8.13
SDA_EXT  (via drill 0.5)
  Top 0.406: v93.98,17.02 93.98,16.76 93.73,16.51 93.73,15.83 U8.P$3
  Bottom 0.254: X2.1 94.74,17.53
  Bottom 0.406: 94.74,17.53 v93.98,17.02
SDA_P0  (via drill 0.5)
  Top 0.254: v42.67,15.49 41.91,15.49 32,5.59 26.42,5.59 25.91,5.08 v25.65,5.33 | v44.96,13.21 44.96,11.94 47.93,8.96 | v17.27,2.29 16.26,3.3 16.26,4.61 U2.1
  Top 0.305: 57.66,20.57 57.4,20.83 57.4,21.34 57.15,21.59
  Top 0.406: I2C-EXT.2 69.85,2.54 68.33,1.02 60.71,1.02 60.33,1.4 R5.1 60.2,4.32 59.44,5.08 v59.18,5.08 | U3.P$3 57.83,20.57 57.66,20.57 | 55.63,22.35 55.63,26.16 55.88,26.42 65.53,26.42 67.97,23.98 U6.13 | PHOTON.13 55.12,13.21 55.12,21.84 55.63,22.35 | 57.15,21.59 56.39,22.35 55.63,22.35
  Top 0.61: PHOTON.13 50.4,11.43 47.93,8.96 J1.P$3-
  Bottom 0.254: v17.27,2.29 16.26,3.3 16.26,3.81 16.76,4.32 24.64,4.32 v25.65,5.33 | v44.96,13.21 v42.67,15.49
  Bottom 0.406: v59.18,5.08 59.18,5.59 PHOTON.13
SDO/ADR
  Top 0.406: R8.1 57.25,23.01 57.4,22.86 59.18,22.86 59.18,22.07 U3.P$5
SS_P0  (via drill 0.5)
  Top 0.406: v78.99,22.86 78.99,22.61 80.01,21.59 MICRO_SD.2 | PHOTON.10 v59.69,27.94
  Bottom 0.406: v78.99,22.86 71.88,22.86 69.34,25.4 62.23,25.4 v59.69,27.94
SYSOFF  (via drill 0.5)
  Top 0.254: v21.59,27.69 21.59,29.72 S1.2 | v25.15,11.68 25.15,10.41 U1.15
  Bottom 0.254: v21.59,27.69 20.83,26.92 20.83,16 v25.15,11.68
TS  (via drill 0.5)
  Top 0.254: U1.1 23.93,9.86 22.86,10.92 v22.61,10.67 | R21.2 11.85,4.99 12.19,5.33 14.48,5.33 14.73,5.59 14.73,8.13 14.99,8.38 15.49,8.38 16,8.89 16,10.16 16.26,10.41 16.26,10.67 16.51,10.92 v17.02,10.92 17.27,10.67 17.27,10.16 17.58,9.85 U2.10
  Top 0.61: R21.2 11.68,3.05 9.4,3.05 8.89,2.54 R24.2
  Bottom 0.254: v22.61,10.67 21.84,11.43 17.53,11.43 v17.02,10.92
V_BATT
  Top 0.254: U2.7 20.38,9.09 20.57,8.89 21.59,8.89 C11.1
  Top 0.279: U1.2 23.11,9.14 22.86,8.89 23.11,8.64 U1.3
  Top 0.61: R1.1 19.82,13.97 18.29,15.49 18.29,19.47 R23.1
  pour Top (isolate 0.203, no thermals): 18.73,13.97 20.7,13.97 20.7,11.56 22.92,9.33 23.5,9.33 23.5,8.51 22.1,8.51 22.1,8.38 21.08,8.38 21.08,9.53 18.73,11.87
V_SOLAR
  Top 1.27: J2.VIN0 16.62,27.18 17.78,27.18 18.29,26.67 19.56,25.4 26.79,18.16 C2.1
  pour Top (isolate 0.203, no thermals): 26.16,10.03 26.16,14.35 26.54,14.73 26.86,14.73 27.56,14.03 27.56,11.81 26.42,10.67 26.42,10.03
VIN_P0  (via drill 0.5)
  Top 0.254: C3.1 27.14,8.9 U1.10 U1.11 | D1.A 24.89,3.3 24.89,3.56 25.65,4.32 25.91,4.32 26.67,5.08 29.97,5.08 | v35.81,7.87 35.31,7.37 34.54,7.37 31.88,4.7 31.5,5.08 29.97,5.08 | D2.A 29.97,5.08
  Top 1.27: PHOTON.1 81.28,31.24 80.77,31.75 38.1,31.75 37.08,30.73 37.08,13.97 34.04,10.92 | 34.04,10.92 v34.04,9.65 | C3.1 29.21,10.92 29.46,11.18 31.46,11.18 R17.1 33.82,11.14 34.04,10.92
  Bottom 0.254: v34.04,9.65 v35.81,7.87
  pour Top (isolate 0.305, no thermals): 27.05,9.27 28.26,9.27 28.38,9.4 29.84,9.4 29.84,8.38 28.32,8.38 28.19,8.51 27.05,8.51

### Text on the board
tPlace: OFF | ON | BATT | V | IN | V | CHG | PWR
bPlace: !PGD! | TS / Disable
tNames: Designed by: pnaylor@gmail.com | BzBox v01 / AKER 2016

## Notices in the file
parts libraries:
SparkFun-Aesthetics: Licensing: Creative Commons ShareAlike 4.0 International - https://creativecommons.org/licenses/by-sa/4.0
SparkFun-Aesthetics: Released under the Creative Commons
SparkFun-Aesthetics: http://creativecommons.org/licenses/by-sa/3.0
